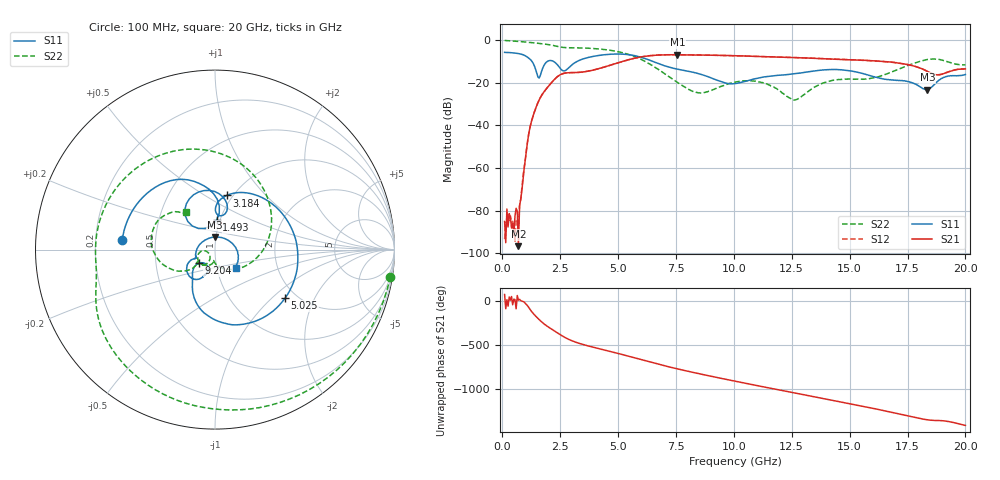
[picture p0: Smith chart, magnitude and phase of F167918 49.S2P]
!  2-Port S-parameters saved by WinCal
! VAR MeasName=S-Parameters (CALIBRATED_DATA) read from VNA (N5242A)
! VAR MeasDate=2016-11-22 10:27:11
! VAR NAME=F167918 49
! VAR FILENAME=F167918 49.S2P
! VAR DATE=2016-11-22 10:27:11
! VAR PHYS_PORTS=1,2
# Hz S DB R 50
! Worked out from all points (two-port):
!   401 points, 100 MHz to 20 GHz, reference 50 ohm
!   highest |S21| = -6.80 dB at 7.562 GHz (marker M1); lowest = -96.6 dB at 697 MHz (marker M2)
!   |S21| within 3 dB of the highest: 5.235 GHz to 16.26 GHz (11.03 GHz wide, 103 % of centre)
!   lowest |S11| = -23.1 dB at 18.36 GHz (marker M3), VSWR 1.15, Z = 49.4 + j6.92 ohm
!   |S11| at or under -10 dB: 1.286 GHz to 1.938 GHz (652.2 MHz wide, 40.5 % of centre); 2.221 GHz to 3.221 GHz (999.1 MHz wide, 36.7 % of centre); 6.52 GHz to end of sweep
!   |S22| runs from -28.1 to -0.1 dB; largest |S21 - S12| = 0.0047
!   S11 on the Smith chart (normalised r, x): 100 MHz: 0.32, +0.05; 1.493 GHz: 0.96, +0.33; 3.184 GHz: 0.94, +0.63; 5.025 GHz: 1.75, -1.22; 9.204 GHz: 0.82, -0.13; 20 GHz: 1.24, -0.26
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1e8  -5.69 174.1  -85.08 78.6  -93.33 34.8  -0.10 -8.8
6.97e8  -6.25 137.1  -96.64 14.4  -88.37 44.5  -0.53 -56.1
1.14475e9  -8.42 103.5  -43.78 -69.4  -43.79 -69.3  -0.99 -87.9
1.493e9  -15.66 86.8  -30.49 179.2  -30.48 179.2  -1.37 -110.0
1.84125e9  -11.08 126.9  -23.63 96.7  -23.61 96.7  -1.82 -130.3
2.33875e9  -11.03 78.1  -17.47 9.6  -17.47 9.6  -2.79 -156.1
2.687e9  -14.38 83.4  -15.46 -47.0  -15.46 -46.9  -3.43 -168.8
3.1845e9  -10.21 77.9  -15.15 -104.8  -15.15 -104.8  -3.55 172.8
3.43325e9  -8.97 63.2  -14.95 -125.7  -14.95 -125.7  -3.61 162.5
5.02525e9  -6.46 -34.6  -10.47 126.7  -10.48 126.7  -5.43 86.5
5.871e9  -7.65 -82.4  -8.08 67.2  -8.05 67.2  -8.38 35.4
6.7665e9  -11.05 -115.4  -6.93 4.1  -6.92 4.1  -13.88 -24.5
7.5625e9  -13.56 -126.7  -6.80 -47.2  -6.79 -47.2  -19.79 -73.4
9.20425e9  -18.46 -140.2  -7.06 -141.7  -7.04 -141.8  -22.72 -98.2
1.005e10  -20.34 -119.7  -7.26 172.4  -7.26 172.4  -19.69 -120.9
1.1642e10  -16.79 -110.7  -7.80 89.3  -7.77 89.2  -21.53 -171.2
1.258725e10  -15.74 -113.4  -8.11 40.8  -8.10 40.8  -28.06 -148.0
1.338325e10  -14.58 -118.4  -8.45 -0.2  -8.40 -0.1  -22.71 -117.5
1.507475e10  -14.43 -146.3  -9.17 -86.6  -9.13 -87.1  -18.31 -142.7
1.67165e10  -18.59 -156.2  -10.17 -176.0  -10.22 -176.1  -15.32 -140.5
1.835825e10  -23.14 90.6  -14.60 92.6  -14.56 92.7  -9.02 176.8
2e10  -16.08 -41.1  -13.45 28.7  -13.39 29.0  -11.56 127.8
